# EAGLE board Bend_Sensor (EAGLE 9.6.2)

No outline drawn. Coordinates in mm, seen from the top.
Copper layers (1*16): Top 0.035mm / dielectric 1.5mm / Bottom 0.035mm
Design rules "default": minimum track width 6mil, minimum drill 0.35mm, track to track 6mil, track to pad 6mil, pad to pad 6mil, via to via 6mil, smd to smd 6mil, copper to edge 40mil, drill to drill 6mil, minimum pad ring 10mil, minimum via ring 8mil, stop-mask expansion 4mil, vias tented up to drill 0mil, thermal gap 10mil

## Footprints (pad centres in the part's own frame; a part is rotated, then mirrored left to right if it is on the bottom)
C369-1 = drill 1.118 long: D 0,-1.397; G -2.286,-1.397; S 2.286,-1.397

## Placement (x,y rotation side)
E$1  [C369-1]  7.62,3.81 0 top

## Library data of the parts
E$1 = transistor-small-signal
